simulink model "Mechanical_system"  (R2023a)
settings: Solver=VariableStepAuto  StartTime=0.0  StopTime=10.0  RelTol=1e-3
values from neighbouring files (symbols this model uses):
  R = 1    [Mechanical_system_EQN.m]    (also in Mechanical_system_SLX_m.m; Electrical_Transformer_EQN.m; Electrical_Transformer_SLX_m.m; Mechanical_Transmission_EQN.m)
undefined symbols (not defined in the file or in its folder): rTm
libraries: fl_lib x10, nesl_utility x2

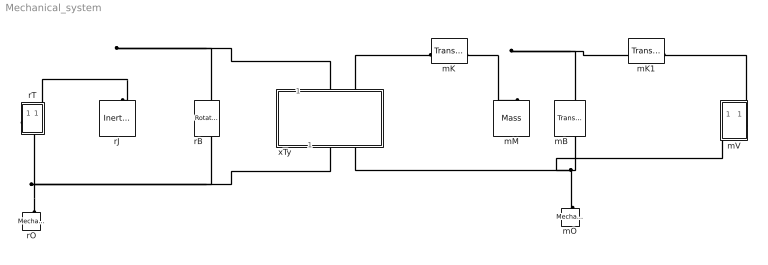
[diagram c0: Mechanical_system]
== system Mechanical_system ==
  mB : fl_lib/Mechanical/Translational Elements/Translational Damper  D=100 N*s/m  v_specify=off  v_priority=None  v=0 m/s  v_nominal_specify=off  v_nominal_unit=m/s  v_nominal_value=1  f_specify=off  f_priority=None  f=0 N  f_nominal_specify=off  f_nominal_unit=N  f_nominal_value=1
  mK : fl_lib/Mechanical/Translational Elements/Translational Spring  spr_rate=1000 N/m  v_specify=off  v_priority=None  v=0 m/s  v_nominal_specify=off  v_nominal_unit=m/s  v_nominal_value=1  f_specify=off  f_priority=None  f=0 N  f_nominal_specify=off  f_nominal_unit=N  f_nominal_value=1  x_specify=off  x_priority=High  x=0 m  x_nominal_specify=off  x_nominal_unit=m  x_nominal_value=1
  mK1 : fl_lib/Mechanical/Translational Elements/Translational Spring  spr_rate=1000 N/m  v_specify=off  v_priority=None  v=0 m/s  v_nominal_specify=off  v_nominal_unit=m/s  v_nominal_value=1  f_specify=off  f_priority=None  f=0 N  f_nominal_specify=off  f_nominal_unit=N  f_nominal_value=1  x_specify=off  x_priority=High  x=0 m  x_nominal_specify=off  x_nominal_unit=m  x_nominal_value=1
  mM : fl_lib/Mechanical/Translational Elements/Mass  mass=1 kg  num_ports=foundation.enum.numPorts2.one  v_specify=off  v_priority=High  v=0 m/s  v_nominal_specify=off  v_nominal_unit=m/s  v_nominal_value=1  f_specify=off  f_priority=None  f=0 N  f_nominal_specify=off  f_nominal_unit=N  f_nominal_value=1
  mO : fl_lib/Mechanical/Translational Elements/Mechanical Translational Reference
  mV : Subsystem  mask{mV='Va'}
      mask prompts: mV "Output variable"
  rB : fl_lib/Mechanical/Rotational Elements/Rotational Damper  D=0.001 N*m*s/rad  w_specify=off  w_priority=None  w=0 rad/s  w_nominal_specify=off  w_nominal_unit=rad/s  w_nominal_value=1  t_specify=off  t_priority=None  t=0 N*m  t_nominal_specify=off  t_nominal_unit=N*m  t_nominal_value=1
  rJ : fl_lib/Mechanical/Rotational Elements/Inertia  inertia=0.01 kg*m^2  num_ports=foundation.enum.numPorts2.one  w_specify=off  w_priority=High  w=0 rad/s  w_nominal_specify=off  w_nominal_unit=rad/s  w_nominal_value=1  t_specify=off  t_priority=None  t=0 N*m  t_nominal_specify=off  t_nominal_unit=N*m  t_nominal_value=1
  rO : fl_lib/Mechanical/Rotational Elements/Mechanical Rotational Reference
  rT : Subsystem  mask{rT='Ta'}
      mask prompts: rT "Output variable"
  xTy : Subsystem  mask{Transformer_type=rTm, T_type=E2=K*E1, xTy=R}
      mask prompts: Transformer_type "Type of Transformer"; T_type "Type of relation"; xTy "Name of parameter K"
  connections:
  rO/LConn1 -- rT/RConn1 -- rB/RConn1 -- xTy/RConn1
  rT/LConn1 -- rB/LConn1 -- xTy/LConn1 -- rJ/LConn1
  xTy/LConn2 -- mK/LConn1
  mK/RConn1 -- mM/LConn1 -- mB/LConn1 -- mK1/LConn1
  xTy/RConn2 -- mV/RConn1 -- mO/LConn1 -- mB/RConn1
  mV/LConn1 -- mK1/RConn1

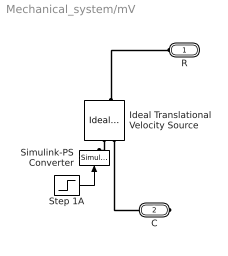
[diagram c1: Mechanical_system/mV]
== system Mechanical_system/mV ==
  Ideal Translational Velocity Source : fl_lib/Mechanical/Mechanical Sources/Ideal Translational Velocity Source
  Simulink-PS Converter : nesl_utility/Simulink-PS Converter  PhysicalDomain=network_engine_domain  SubClassName=ps_input  LeftPortType=input  RightPortType=output  PseudoPeriodic=off  Frequencies=[]  NoiseDistribution=none  NoiseParameters=[]  Unit=1  AffineConversion=off  FilteringAndDerivatives=zero  SimscapeFilterOrder=1  InputFilterTimeConstant=.001  UdotUserProvided=0
  Step 1A : Step  After=100  SampleTime=0
  R : PMIOPort  Side=Left
  C : PMIOPort  Port=2  Side=Right
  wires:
  Step 1A/1 -> Simulink-PS Converter/1
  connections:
  Ideal Translational Velocity Source/RConn1 -- Simulink-PS Converter/RConn1
  Ideal Translational Velocity Source/LConn1 -- R/RConn1
  Ideal Translational Velocity Source/RConn2 -- C/RConn1

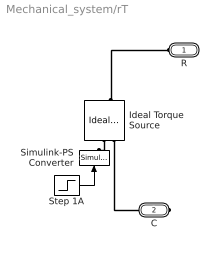
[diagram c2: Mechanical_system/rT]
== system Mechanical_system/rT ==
  Ideal Torque Source : fl_lib/Mechanical/Mechanical Sources/Ideal Torque Source
  Simulink-PS Converter : nesl_utility/Simulink-PS Converter  PhysicalDomain=network_engine_domain  SubClassName=ps_input  LeftPortType=input  RightPortType=output  PseudoPeriodic=off  Frequencies=[]  NoiseDistribution=none  NoiseParameters=[]  Unit=1  AffineConversion=off  FilteringAndDerivatives=zero  SimscapeFilterOrder=1  InputFilterTimeConstant=.001  UdotUserProvided=0
  Step 1A : Step  After=100  SampleTime=0
  R : PMIOPort  Side=Left
  C : PMIOPort  Port=2  Side=Right
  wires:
  Step 1A/1 -> Simulink-PS Converter/1
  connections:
  Ideal Torque Source/RConn2 -- C/RConn1
  Ideal Torque Source/LConn1 -- R/RConn1
  Ideal Torque Source/RConn1 -- Simulink-PS Converter/RConn1

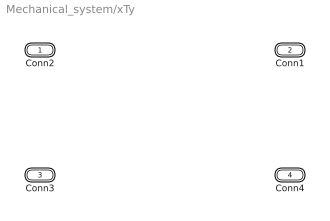
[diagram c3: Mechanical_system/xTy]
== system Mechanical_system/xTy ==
  Conn2 : PMIOPort  Side=Left
  Conn1 : PMIOPort  Port=2  Side=Left
  Conn3 : PMIOPort  Port=3  Side=Right
  Conn4 : PMIOPort  Port=4  Side=Right
